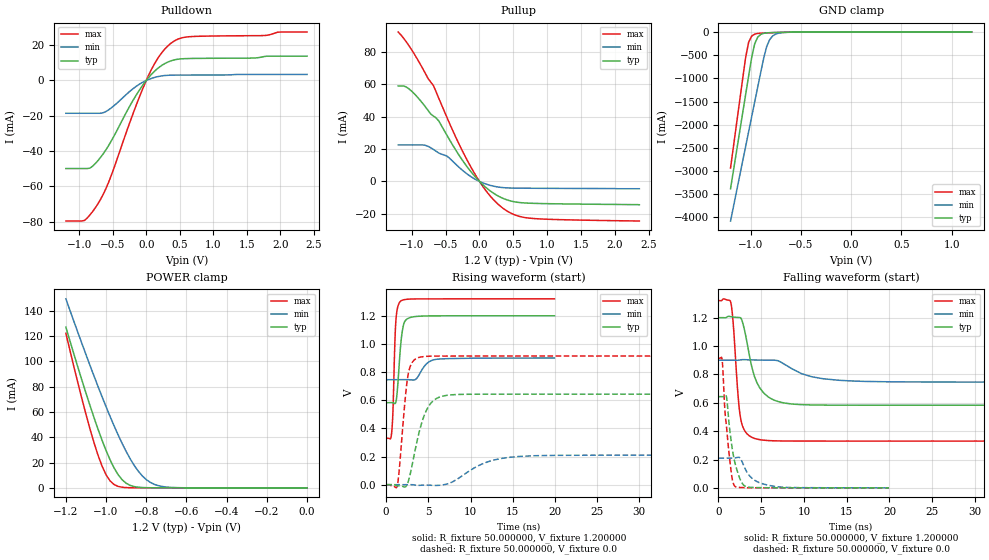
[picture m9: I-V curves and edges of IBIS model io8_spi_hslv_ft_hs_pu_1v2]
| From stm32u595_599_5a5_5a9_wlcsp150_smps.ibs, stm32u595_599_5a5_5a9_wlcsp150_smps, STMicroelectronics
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|   Model io8_spi_hslv_ft_hs_pu_1v2
[Model]  io8_spi_hslv_ft_hs_pu_1v2
Model_type I/O
Polarity   Non-Inverting
Enable   Active-Low
Vinl =   0.360000V
Vinh =   0.840000V
Vmeas =  0.600000V
Cref =   50.000000pF
Rref =   100.000000M
Vref =   0.0V
C_comp   3.133100pF   3.070300pF   3.178200pF
[Temperature Range]   25.000000   0.140000k   -40.000000
[Pullup Reference]   1.200000V   0.900000V   1.320000V
[Pulldown Reference]   0.0V   0.0V   0.0V
[POWER Clamp Reference]   1.200000V   0.900000V   1.320000V
[GND Clamp Reference]   0.0V   0.0V   0.0V
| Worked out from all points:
|   slope of the pulldown table from 0 to 0.18 V, typ, clamps not added: 25.4 ohm
|   slope of the pullup table from 0 to 0.18 V, typ, clamps not added: 27.8 ohm
|   GND clamp passes 1 mA (typ) near -0.51 V on its own axis
|   POWER clamp passes 1 mA (typ) near -0.86 V on its own axis
|   rising waveform, R_fixture 50.000000, V_fixture 1.200000: 20-80 % time 503ps typ, 1.13ns min, 303ps max; typ from 0.583 V to 1.2 V
|   rising waveform, R_fixture 50.000000, V_fixture 0.0: 20-80 % time 1.63ns typ, 3.83ns min, 811ps max; typ from 0 V to 0.643 V
|   falling waveform, R_fixture 50.000000, V_fixture 1.200000: 20-80 % time 1.65ns typ, 3.75ns min, 725ps max; typ from 1.2 V to 0.583 V
|   falling waveform, R_fixture 50.000000, V_fixture 0.0: 20-80 % time 1ns typ, 1.7ns min, 754ps max; typ from 0.643 V to 0 V
[Pulldown]
|Voltage   I(typ)   I(min)   I(max)
-1.2V     -49.85mA   -18.57mA   -79.56mA
-920mV    -49.85mA   -18.57mA   -79.19mA
-840mV    -49.59mA   -18.57mA   -76.08mA
-720mV    -45.32mA   -18.57mA   -69.73mA
-560mV    -36.71mA   -16.58mA   -57.44mA
-200mV    -11.43mA   -4.74mA    -19.03mA
0V        0A         0A         0A
160mV     6.476mA    2.075mA    11.78mA
360mV     10.99mA    2.989mA    20.81mA
480mV     12.07mA    3.053mA    23.52mA
640mV     12.42mA    3.074mA    24.76mA
2.4V      13.77mA    3.423mA    27.42mA
[Pullup]
|Voltage   I(typ)   I(min)   I(max)
-1.2V     59.07mA    22.59mA    92.4mA
-1V       55.77mA    22.59mA    81.31mA
-800mV    46.22mA    22.35mA    66.88mA
-680mV    40.45mA    19.8mA     59.31mA
-600mV    37.33mA    17.55mA    51.34mA
-320mV    17.39mA    9.466mA    24.7mA
-80mV     3.667mA    1.75mA     5.47mA
120mV     -4.592mA   -1.936mA   -7.077mA
320mV     -9.941mA   -3.694mA   -15.72mA
520mV     -12.61mA   -4.111mA   -20.65mA
760mV     -13.48mA   -4.204mA   -22.78mA
2.36V     -14.4mA    -4.5mA     -24.46mA
[GND_clamp]
|Voltage   I(typ)   I(min)   I(max)
-1.2V     -3.379A    -4.076A    -2.932A
-1.05V    -1.35A     -2.47A     -550.7mA
-1.02V    -947.8mA   -2.149A    -221.5mA
-990mV    -552.4mA   -1.829A    -88.44mA
-960mV    -255.3mA   -1.51A     -44.87mA
-930mV    -111.8mA   -1.191A    -30.68mA
-870mV    -28.35mA   -564.6mA   -21.34mA
-840mV    -18.65mA   -309.5mA   -18.49mA
-810mV    -14.07mA   -161.6mA   -15.92mA
-780mV    -11.37mA   -83.33mA   -13.53mA
-600mV    -3.009mA   -4.321mA   -3.091mA
1.2V      0A         13.65nA    0A
[POWER_clamp]
|Voltage   I(typ)   I(min)   I(max)
-1.2V     127mA      149.4mA    122.2mA
-1.12V    84.98mA    114mA      70.29mA
-1.06V    55.52mA    88.42mA    35.69mA
-1.02V    37.64mA    72.04mA    17.19mA
-1V       29.52mA    64.13mA    10.33mA
-960mV    15.7mA     48.99mA    2.596mA
-900mV    3.636mA    28.77mA    207.8uA
-840mV    502.9uA    13.24mA    43.46uA
-800mV    129uA      6.535mA    43.46uA
-740mV    26.25uA    1.726mA    43.46uA
-620mV    25.09uA    82.33uA    35.76uA
0V        0A         17.36nA    0A
[Ramp]
| variable   typ   min   max
dV/dt_r  0.38570/1.62823n   0.12567/3.82967n   0.54818/0.80593n
dV/dt_f  0.37036/1.64180n   92.35200m/3.75123n  0.59402/0.72107n
R_load = 50.000000
[Rising Waveform]
R_fixture= 50.000000
V_fixture= 1.200000
V_fixture_min= 0.900000
V_fixture_max= 1.320000
|time   V(typ)   V(min)   V(max)
0s        582.8mV    746.1mV    330.1mV
640.6ps   583.1mV    746.1mV    363.9mV
800.8ps   581.8mV    746.1mV    516.7mV
1.041ns   576mV      746.1mV    1.028V
1.161ns   589.8mV    746.1mV    1.172V
1.722ns   993.5mV    746.2mV    1.304V
2.162ns   1.155V     746.3mV    1.315V
3.083ns   1.191V     744.2mV    1.319V
5.886ns   1.2V       890.5mV    1.32V
19.94ns   1.2V       900mV      1.32V
[Rising Waveform]
R_fixture= 50.000000
V_fixture= 0.0
V_fixture_min= 0.0
V_fixture_max= 0.0
|time   V(typ)   V(min)   V(max)
0s        431.2uV    496.5uV    357.3uV
1.301ns   -8.037mV   488.4uV    -13.35mV
2.302ns   -14.56mV   530.5uV    638.9mV
2.603ns   20.09mV    632.1uV    782.5mV
3.804ns   347.2mV    -4.328mV   902.5mV
5.205ns   572.2mV    -3.304mV   912.9mV
7.407ns   636.5mV    9.212mV    913.9mV
11.51ns   643mV      151mV      914.1mV
15.72ns   643.3mV    200.9mV    914.1mV
49.85ns   643.4mV    210mV      914.1mV
[Falling Waveform]
R_fixture= 50.000000
V_fixture= 1.200000
V_fixture_min= 0.900000
V_fixture_max= 1.320000
|time   V(typ)   V(min)   V(max)
0s        1.2V       900mV      1.32V
1.401ns   1.208V     900mV      1.316V
1.702ns   1.204V     900mV      1.175V
2.302ns   1.202V     899.9mV    640.9mV
2.603ns   1.198V     902.6mV    485mV
4.204ns   786mV      901.7mV    349.3mV
5.806ns   642mV      900.6mV    333.8mV
9.009ns   589.4mV    826.8mV    330.3mV
16.72ns   582.8mV    751.5mV    330.1mV
49.85ns   582.8mV    746.1mV    330.1mV
[Falling Waveform]
R_fixture= 50.000000
V_fixture= 0.0
V_fixture_min= 0.0
V_fixture_max= 0.0
|time   V(typ)   V(min)   V(max)
0s        643.4mV    210mV      914.1mV
440.4ps   643.2mV    210mV      895.8mV
720.7ps   647.9mV    210.1mV    572.6mV
920.9ps   645.4mV    210.1mV    443.8mV
1.522ns   313.6mV    209.9mV    96.17mV
1.922ns   178.1mV    211mV      11.22mV
2.643ns   46.18mV    199.1mV    2.634mV
3.443ns   5.36mV     100.2mV    1.159mV
6.887ns   668.8uV    8.225mV    374.7uV
19.94ns   431.2uV    496.5uV    357.3uV
